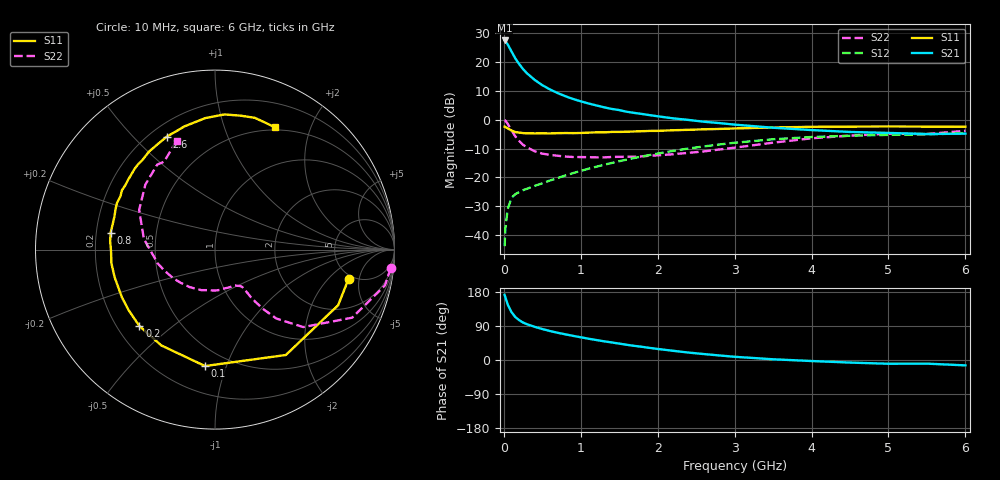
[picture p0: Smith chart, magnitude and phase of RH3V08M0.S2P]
! SIEMENS Small Signal Semiconductors
! BFR106
! Si NPN RF Bipolar Junction Transistor in SOT23
! VCE = 3 V  IC = 8 mA
! Common Emitter S-Parameters:  August  1996
# GHz  S  MA  R  50
!  f  S11  S21  S12  S22
! GHz  MAG  ANG  MAG  ANG  MAG  ANG  MAG  ANG
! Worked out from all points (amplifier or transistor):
!   36 points, 10 MHz to 6 GHz, reference 50 ohm
!   highest |S21| = 27.5 dB at 10 MHz (marker M1)
!   |S21| within 3 dB of that: start of sweep to 82.97 MHz
!   unconditionally stable (mu >= 1): 517 MHz to 2.126 GHz; 4.872 GHz to end of sweep
!   at 250 MHz: K = 0.65, MSG = 21.0 dB, |S12| = -24.4 dB
!   at 1.4 GHz: K = 1.11, MAG = 7.4 dB, |S12| = -15.0 dB
!   at 6 GHz: K = 1.02, MAG = -0.9 dB, |S12| = -4.7 dB
!   S11 on the Smith chart (normalised r, x): 10 MHz: 4.58, -3.54; 100 MHz: 0.38, -0.85; 200 MHz: 0.29, -0.39; 800 MHz: 0.26, +0.08; 2.6 GHz: 0.27, +0.63; 6 GHz: 0.46, +1.50
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0.01  0.7618 -12.3  23.82 172.0  0.0064 84.0  0.9848 -6.0
0.02  0.7528 -24.3  23.18 165.6  0.0131 77.3  0.9679 -11.9
0.05  0.7075 -56.1  20.3 146.6  0.0283 64.2  0.8531 -26.4
0.1  0.6511 -94.9  15.32 126.2  0.0443 50.9  0.654 -41.3
0.15  0.612 -119.2  11.57 113.0  0.0512 44.7  0.5145 -48.3
0.2  0.5991 -134.6  9.257 105.1  0.0558 42.8  0.4283 -50.9
0.25  0.5876 -145.2  7.579 98.8  0.06 42.8  0.367 -52.3
0.3  0.5827 -152.9  6.42 94.6  0.0634 44.1  0.3327 -53.0
0.4  0.5801 -164.6  4.935 87.6  0.0713 46.7  0.2844 -53.3
0.5  0.5821 -172.5  3.985 81.7  0.0789 50.0  0.2584 -53.9
0.6  0.5795 -179.4  3.358 76.5  0.0883 52.4  0.246 -55.5
0.7  0.5862 175.3  2.91 71.8  0.0975 54.6  0.2374 -58.1
0.8  0.5891 170.7  2.56 67.7  0.108 56.3  0.23 -60.6
1.1  0.5983 157.8  1.92 56.2  0.1413 59.2  0.2243 -71.2
1.3  0.6045 150.7  1.651 49.4  0.1655 59.7  0.2224 -79.2
1.6  0.6212 141.1  1.377 40.1  0.2039 58.8  0.2283 -93.3
2.2  0.6581 124.0  1.06 24.3  0.2883 53.4  0.2525 -124.2
2.6  0.6843 113.1  0.925 15.7  0.3446 47.8  0.2827 -146.1
3.5  0.7348 94.2  0.728 1.9  0.4595 32.6  0.4005 171.5
4.5  0.7598 79.1  0.615 -6.8  0.5286 15.1  0.5307 137.0
5.5  0.76 67.7  0.566 -9.6  0.5573 4.1  0.5664 120.0
6  0.7593 64.0  0.575 -14.2  0.5839 -3.6  0.6429 109.4
